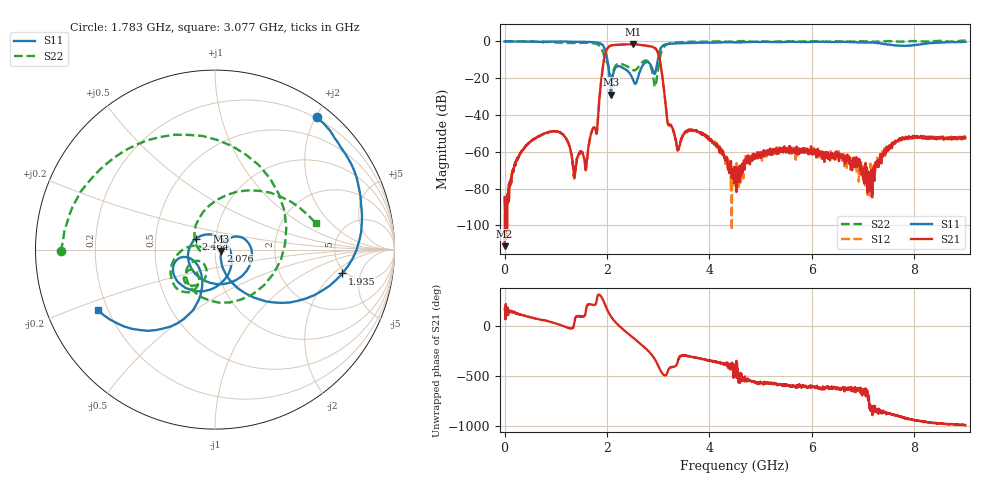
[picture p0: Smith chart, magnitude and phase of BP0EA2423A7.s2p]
!Agilent Technologies,E8358A,US40260310,A.06.04.32
!Agilent E8358A: A.06.04.32
!Date: Tuesday, September 01, 2020 10:49:37
!Correction: S11(Full 2 Port(1,2)) S21(Full 2 Port(1,2)) S12(Full 2 Port(1,2)) S22(Full 2 Port(1,2))
!S2P File: Measurements: S11, S21, S12, S22:
# Hz S  dB  R 50
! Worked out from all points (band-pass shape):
!   1601 points, 300 kHz to 9 GHz, reference 50 ohm
!   highest |S21| = -1.56 dB at 2.509 GHz (marker M1); lowest = -111.3 dB at 300 kHz (marker M2)
!   |S21| within 3 dB of the highest: 1.994 GHz to 2.966 GHz (972.3 MHz wide, 39.2 % of centre)
!   lowest |S11| = -28.9 dB at 2.076 GHz (marker M3), VSWR 1.07, Z = 53.6 - j0.833 ohm
!   |S11| at or under -10 dB: 2.007 GHz to 2.991 GHz (984 MHz wide, 39.4 % of centre)
!   |S22| runs from -24.7 to 0.5 dB; largest |S21 - S12| = 0.0061
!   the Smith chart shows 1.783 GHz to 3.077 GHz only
!   S11 on the Smith chart (normalised r, x): 1.783 GHz: 0.19, +2.01; 1.935 GHz: 4.70, -2.62; 2.076 GHz: 1.07, -0.02; 2.464 GHz: 0.80, +0.10; 3.077 GHz: 0.16, -0.24
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300000  -0.02 -180.0  -111.30 171.9  -83.91 143.2  -0.00 -0.3
2.590414e8  -0.10 169.4  -63.59 125.8  -63.13 123.4  0.09 -87.5
6.021549e8  -0.25 155.7  -52.57 80.7  -52.80 79.6  -0.20 -166.4
1.06339e9  -0.09 132.3  -49.18 20.2  -49.26 19.9  -0.75 85.5
1.282757e9  -0.17 116.9  -58.35 -20.8  -58.40 -17.8  -0.94 1.2
1.502125e9  -0.31 97.3  -59.91 99.6  -60.11 101.1  -0.75 -82.3
1.783366e9  -0.63 52.5  -48.73 -130.7  -48.86 -130.4  -1.34 -179.3
1.935236e9  -2.82 -10.6  -10.97 -107.9  -10.96 -107.6  -7.06 29.2
2.075856e9  -28.90 -12.5  -2.32 101.6  -2.31 101.8  -19.83 -135.4
2.250225e9  -13.58 -46.9  -1.82 -0.5  -1.82 -0.4  -12.12 -131.4
2.463968e9  -18.23 150.8  -1.56 -93.5  -1.57 -93.4  -14.85 -141.1
2.508966e9  -20.95 109.2  -1.56 -112.3  -1.58 -112.3  -15.61 -136.4
2.823956e9  -11.78 -155.7  -2.61 104.8  -2.62 105.0  -11.73 -159.7
3.00395e9  -8.12 -112.2  -6.94 -38.4  -6.92 -38.5  -14.22 117.5
3.077072e9  -2.68 -152.9  -18.22 -110.2  -18.31 -109.9  -4.71 14.6
3.493309e9  -0.98 83.9  -50.70 68.7  -50.26 69.0  -0.40 -103.4
4.50015e9  -0.57 -64.4  -68.22 -122.4  -70.19 -89.5  -0.12 -149.5
6.001975e9  -0.29 -161.3  -60.93 120.1  -59.77 111.0  -0.08 -176.3
7.155062e9  -0.77 133.0  -76.34 -78.1  -74.63 -70.7  -0.10 154.4
7.5038e9  -1.71 85.4  -57.05 -156.4  -57.68 -151.0  0.04 149.0
8.156278e9  -1.46 -75.1  -52.01 125.4  -51.60 125.3  -0.11 142.7
9e9  -0.27 -139.8  -52.76 88.5  -51.91 88.5  0.43 140.9
